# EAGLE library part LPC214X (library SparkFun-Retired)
NXP LPC2144/2146/2148 ARM7 MCU FLASH 512K 64LQFP Datasheet SparkFun Products SparkFun Logomatic v2 - Serial SD Datalogger (FAT32) (WIG-12772)
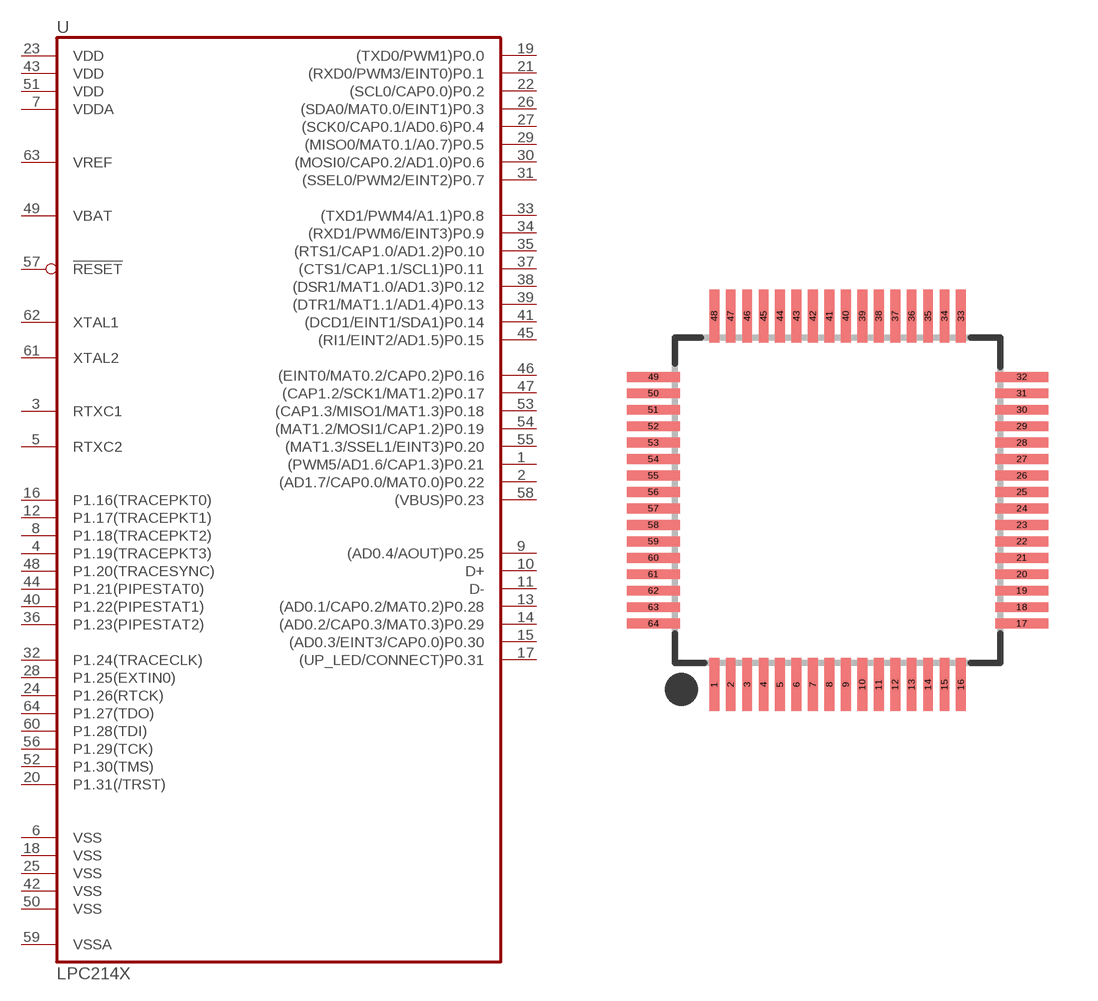
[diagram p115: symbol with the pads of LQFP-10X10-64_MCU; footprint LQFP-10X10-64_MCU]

Designator prefix U

## LPC214X (PROD_ID: IC-07934; VALUE: LPC2148)  [LQFP-10X10-64_MCU]
1  (PWM5/AD1.6/CAP1.3)P0.21
2  (AD1.7/CAP0.0/MAT0.0)P0.22
3  RTXC1  in
4  P1.19(TRACEPKT3)
5  RTXC2  out
6  VSS  pwr
7  VDDA  pwr
8  P1.18(TRACEPKT2)
9  (AD0.4/AOUT)P0.25
10  D+
11  D-
12  P1.17(TRACEPKT1)
13  (AD0.1/CAP0.2/MAT0.2)P0.28
14  (AD0.2/CAP0.3/MAT0.3)P0.29
15  (AD0.3/EINT3/CAP0.0)P0.30
16  P1.16(TRACEPKT0)
17  (UP_LED/CONNECT)P0.31
18  VSS  pwr
19  (TXD0/PWM1)P0.0
20  P1.31(/TRST)
21  (RXD0/PWM3/EINT0)P0.1
22  (SCL0/CAP0.0)P0.2
23  VDD  pwr
24  P1.26(RTCK)
25  VSS  pwr
26  (SDA0/MAT0.0/EINT1)P0.3
27  (SCK0/CAP0.1/AD0.6)P0.4
28  P1.25(EXTIN0)
29  (MISO0/MAT0.1/A0.7)P0.5
30  (MOSI0/CAP0.2/AD1.0)P0.6
31  (SSEL0/PWM2/EINT2)P0.7
32  P1.24(TRACECLK)
33  (TXD1/PWM4/A1.1)P0.8
34  (RXD1/PWM6/EINT3)P0.9
35  (RTS1/CAP1.0/AD1.2)P0.10
36  P1.23(PIPESTAT2)
37  (CTS1/CAP1.1/SCL1)P0.11
38  (DSR1/MAT1.0/AD1.3)P0.12
39  (DTR1/MAT1.1/AD1.4)P0.13
40  P1.22(PIPESTAT1)
41  (DCD1/EINT1/SDA1)P0.14
42  VSS  pwr
43  VDD  pwr
44  P1.21(PIPESTAT0)
45  (RI1/EINT2/AD1.5)P0.15
46  (EINT0/MAT0.2/CAP0.2)P0.16
47  (CAP1.2/SCK1/MAT1.2)P0.17
48  P1.20(TRACESYNC)
49  VBAT  pwr
50  VSS  pwr
51  VDD  pwr
52  P1.30(TMS)
53  (CAP1.3/MISO1/MAT1.3)P0.18
54  (MAT1.2/MOSI1/CAP1.2)P0.19
55  (MAT1.3/SSEL1/EINT3)P0.20
56  P1.29(TCK)
57  !RESET  in
58  (VBUS)P0.23
59  VSSA  pwr
60  P1.28(TDI)
61  XTAL2  out
62  XTAL1  in
63  VREF  in
64  P1.27(TDO)

## Footprint LQFP-10X10-64_MCU (pad centres in mm)
LQFP64 shrink quad flat pack, square
smd 0.3 x 1.6: 1 -3.75,-5.6; 2 -3.25,-5.6; 3 -2.75,-5.6; 4 -2.25,-5.6; 5 -1.75,-5.6; 6 -1.25,-5.6; 7 -0.75,-5.6; 8 -0.25,-5.6; 9 0.25,-5.6; 10 0.75,-5.6; 11 1.25,-5.6; 12 1.75,-5.6; 13 2.25,-5.6; 14 2.75,-5.6; 15 3.25,-5.6; 16 3.75,-5.6; 33 3.75,5.6; 34 3.25,5.6; 35 2.75,5.6; 36 2.25,5.6; 37 1.75,5.6; 38 1.25,5.6; 39 0.75,5.6; 40 0.25,5.6; 41 -0.25,5.6; 42 -0.75,5.6; 43 -1.25,5.6; 44 -1.75,5.6; 45 -2.25,5.6; 46 -2.75,5.6; 47 -3.25,5.6; 48 -3.75,5.6
smd 1.6 x 0.3: 17 5.6,-3.75; 18 5.6,-3.25; 19 5.6,-2.75; 20 5.6,-2.25; 21 5.6,-1.75; 22 5.6,-1.25; 23 5.6,-0.75; 24 5.6,-0.25; 25 5.6,0.25; 26 5.6,0.75; 27 5.6,1.25; 28 5.6,1.75; 29 5.6,2.25; 30 5.6,2.75; 31 5.6,3.25; 32 5.6,3.75; 49 -5.6,3.75; 50 -5.6,3.25; 51 -5.6,2.75; 52 -5.6,2.25; 53 -5.6,1.75; 54 -5.6,1.25; 55 -5.6,0.75; 56 -5.6,0.25; 57 -5.6,-0.25; 58 -5.6,-0.75; 59 -5.6,-1.25; 60 -5.6,-1.75; 61 -5.6,-2.25; 62 -5.6,-2.75; 63 -5.6,-3.25; 64 -5.6,-3.75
